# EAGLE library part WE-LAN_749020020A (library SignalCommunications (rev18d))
LAN-Transformer WE-LAN 10/100/1000 Base Tx - Compliant with IEEE 802.3 standards - SMD -- Ethernet -- Power over Ethernet -- 1 Gigabit Ethernet -- Compliant with most IC's for ethernet applications like Intel, AMD, Globespan and Realtek -- Hub, Router, Switch Details see: http://katalog.we-online.de/en/pbs/WE-LAN/S/749020020A? Updated by Dan Xu 2014-07-08 2014 (C) Würth Elektronik
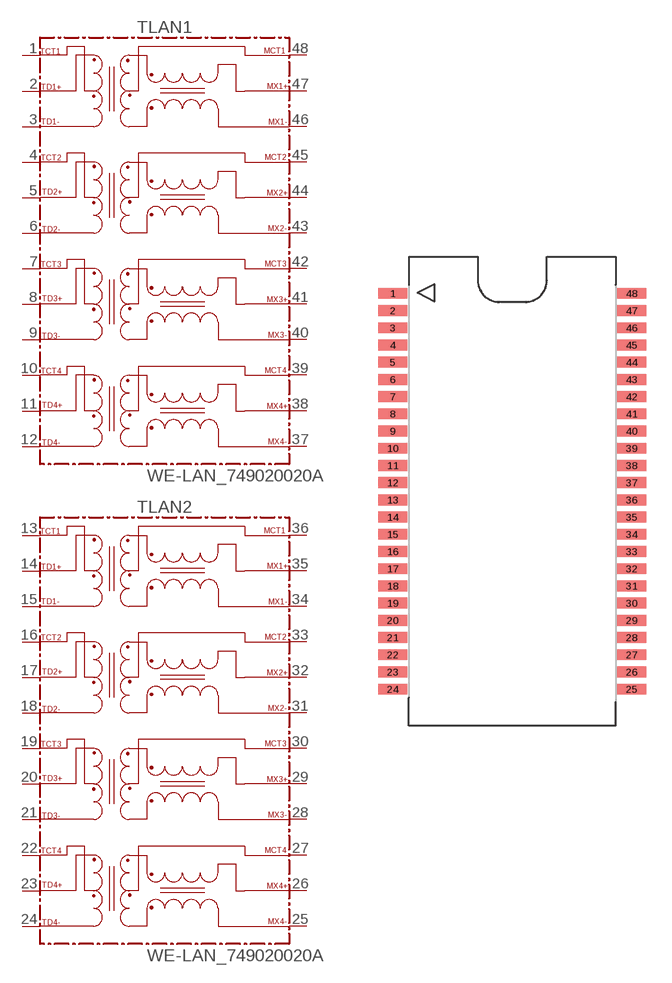
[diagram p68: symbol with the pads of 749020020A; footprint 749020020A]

Designator prefix T; gates LAN1=749020020A LAN2=749020020A

## WE-LAN_749020020A  [749020020A]
1  LAN1:TCT1
2  LAN1:TD1+
3  LAN1:TD1-
4  LAN1:TCT2
5  LAN1:TD2+
6  LAN1:TD2-
7  LAN1:TCT3
8  LAN1:TD3+
9  LAN1:TD3-
10  LAN1:TCT4
11  LAN1:TD4+
12  LAN1:TD4-
13  LAN2:TCT1
14  LAN2:TD1+
15  LAN2:TD1-
16  LAN2:TCT2
17  LAN2:TD2+
18  LAN2:TD2-
19  LAN2:TCT3
20  LAN2:TD3+
21  LAN2:TD3-
22  LAN2:TCT4
23  LAN2:TD4+
24  LAN2:TD4-
25  LAN2:MX4-
26  LAN2:MX4+
27  LAN2:MCT4
28  LAN2:MX3-
29  LAN2:MX3+
30  LAN2:MCT3
31  LAN2:MX2-
32  LAN2:MX2+
33  LAN2:MCT2
34  LAN2:MX1-
35  LAN2:MX1+
36  LAN2:MCT1
37  LAN1:MX4-
38  LAN1:MX4+
39  LAN1:MCT4
40  LAN1:MX3-
41  LAN1:MX3+
42  LAN1:MCT3
43  LAN1:MX2-
44  LAN1:MX2+
45  LAN1:MCT2
46  LAN1:MX1-
47  LAN1:MX1+
48  LAN1:MCT1

## Footprint 749020020A (pad centres in mm)
MAX Height = 7.70mm
smd 1.72 x 0.64: 1 -7.08,11.73; 2 -7.08,10.71; 3 -7.08,9.69; 4 -7.08,8.67; 5 -7.08,7.65; 6 -7.08,6.63; 7 -7.08,5.61; 8 -7.08,4.59; 9 -7.08,3.57; 10 -7.08,2.55; 11 -7.08,1.53; 12 -7.08,0.51; 13 -7.08,-0.51; 14 -7.08,-1.53; 15 -7.08,-2.55; 16 -7.08,-3.57; 17 -7.08,-4.59; 18 -7.08,-5.61; 19 -7.08,-6.63; 20 -7.08,-7.65; 21 -7.08,-8.67; 22 -7.08,-9.69; 23 -7.08,-10.71; 24 -7.08,-11.73; 25 7.08,-11.73; 26 7.08,-10.71; 27 7.08,-9.69; 28 7.08,-8.67; 29 7.08,-7.65; 30 7.08,-6.63; 31 7.08,-5.61; 32 7.08,-4.59; 33 7.08,-3.57; 34 7.08,-2.55; 35 7.08,-1.53; 36 7.08,-0.51; 37 7.08,0.51; 38 7.08,1.53; 39 7.08,2.55; 40 7.08,3.57; 41 7.08,4.59; 42 7.08,5.61; 43 7.08,6.63; 44 7.08,7.65; 45 7.08,8.67; 46 7.08,9.69; 47 7.08,10.71; 48 7.08,11.73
